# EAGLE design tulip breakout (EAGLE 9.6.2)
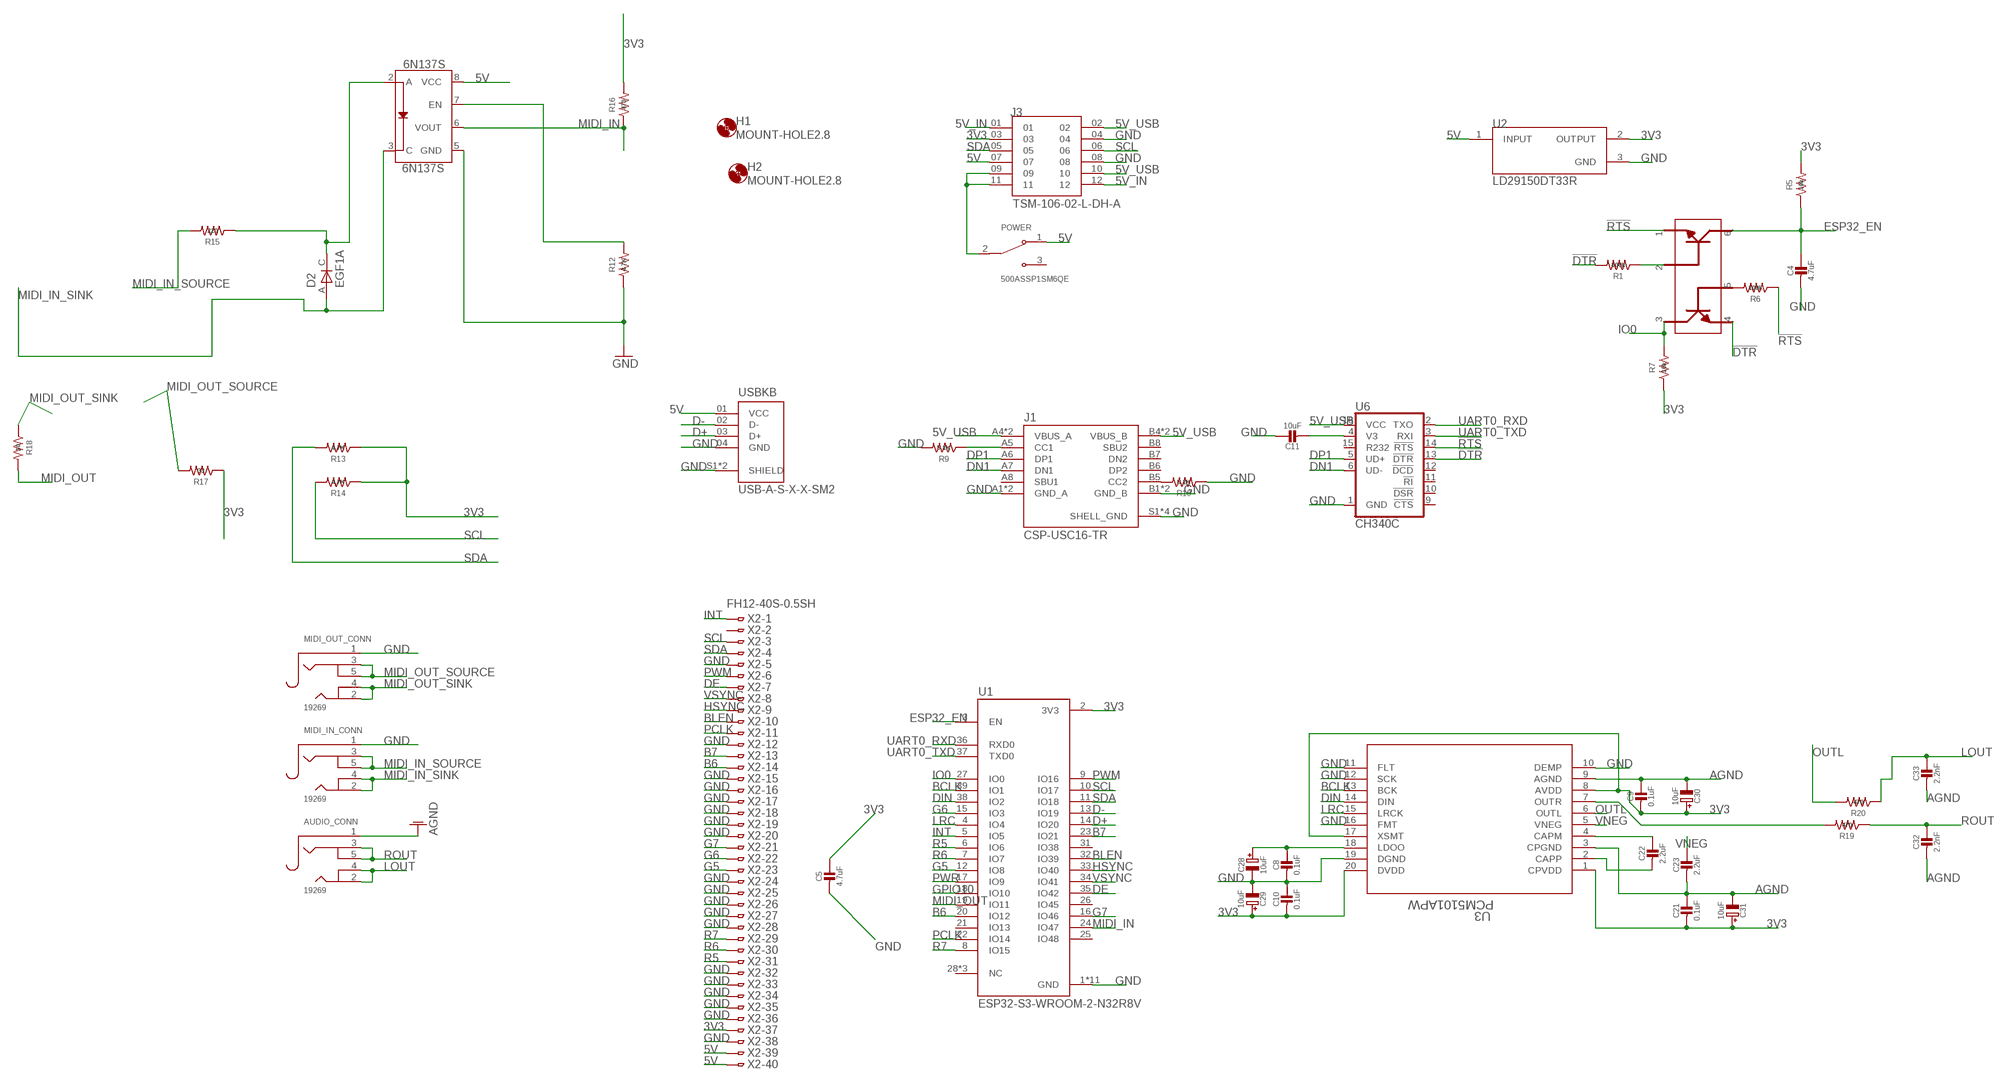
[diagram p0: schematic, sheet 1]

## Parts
6N137S  6N137S  [8-SMD]
AUDIO_CONN  19269  AUDIO_3.5MMJACK  [4UCONN_19269]
C4  4.7uF  CAP_CERAMIC0805-NOOUTLINE  [0805-NO]
C5  4.7uF  CAP_CERAMIC0805-NOOUTLINE  [0805-NO]
C8  0.1uF  CAP_CERAMIC0805-NOOUTLINE  [0805-NO]
C9  0.1uF  CAP_CERAMIC0805-NOOUTLINE  [0805-NO]
C10  0.1uF  CAP_CERAMIC0805-NOOUTLINE  [0805-NO]
C11  10uF  CAP_CERAMIC0805-NOOUTLINE  [0805-NO]
C21  0.1uF  CAP_CERAMIC0805-NOOUTLINE  [0805-NO]
C22  2.2uF  CAP_CERAMIC0805-NOOUTLINE  [0805-NO]
C23  2.2uF  CAP_CERAMIC0805-NOOUTLINE  [0805-NO]
C28  10uF  CAP_ELECTROLYTICPANASONIC_C  [PANASONIC_C]
C29  10uF  CAP_ELECTROLYTICPANASONIC_C  [PANASONIC_C]
C30  10uF  CAP_ELECTROLYTICPANASONIC_C  [PANASONIC_C]
C31  10uF  CAP_ELECTROLYTICPANASONIC_C  [PANASONIC_C]
C32  2.2nF  CAP_CERAMIC0805-NOOUTLINE  [0805-NO]
C33  2.2nF  CAP_CERAMIC0805-NOOUTLINE  [0805-NO]
D2  EGF1A  [DIOM449X264X300L114X135N]
H1  MOUNT-HOLE2.8  [2,8]
H2  MOUNT-HOLE2.8  [2,8]
J1  CSP-USC16-TR  [VALCON_CSP-USC16-TR]
J3  TSM-106-02-L-DH-A  [SAMTEC_TSM-106-02-L-DH-A]
MIDI_IN_CONN  19269  AUDIO_3.5MMJACK  [4UCONN_19269]
MIDI_OUT_CONN  19269  AUDIO_3.5MMJACK  [4UCONN_19269]
POWER  500ASSP1SM6QE  [SW_500ASSP1SM6QE]
R1  100k  R-US_R0805  [R0805]
R5  10k  R-US_R0805  [R0805]
R6  100k  R-US_R0805  [R0805]
R7  10k  R-US_R0805  [R0805]
R9  5.1K  R-US_R0805  [R0805]
R10  5.1K  R-US_R0805  [R0805]
R12  4.7K  R-US_R0805  [R0805]
R13  4.7K  R-US_R0805  [R0805]
R14  4.7K  R-US_R0805  [R0805]
R15  220  R-US_R0805  [R0805]
R16  470  R-US_R0805  [R0805]
R17  33  R-US_R0805  [R0805]
R18  10  R-US_R0805  [R0805]
R19  470  R-US_R0805  [R0805]
R20  470  R-US_R0805  [R0805]
RESET  MBT3904DW1T1G  [SOT236]
U1  ESP32-S3-WROOM-2-N32R8V  [XCVR_ESP32-S3-WROOM-2-N32R8V]
U2  LD29150DT33R  [DPAK456P972X240-3N]
U3  PCM5101APW  [PW20_TEX]
U6  CH340C  [SO016]
USBKB  USB-A-S-X-X-SM2  [SAMTEC_USB-A-S-X-X-SM2]
X2  FH12-40S-0.5SH  [FH12-40S-0.5SH]

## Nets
3V3: C5.1 C9.2 C10.2 C21.2 C29.+ C30.+ C31.+ J3.03 R5.2 R7.1 R13.1 R14.1 R16.2 R17.1 U1.2(3V3) U2.2(OUTPUT) U3.1(CPVDD) U3.8(AVDD) U3.17(XSMT) U3.20(DVDD) X2.37
5V: 6N137S.8(VCC) J3.07 POWER.1(NC) U2.1(INPUT) USBKB.01(VCC) X2.39 X2.40
5V_IN: J3.01 J3.12
5V_USB: J1.A4(VBUS_A) J1.A9(VBUS_A) J1.B4(VBUS_B) J1.B9(VBUS_B) J3.02 J3.10 U6.16(VCC)
!DTR: R1.2 RESET.4 U6.13(!DTR)
!RTS: R6.1 RESET.1 U6.14(!RTS)
AGND: AUDIO_CONN.1 C9.1 C21.1 C23.2 C30.- C31.- C32.2 C33.2 U3.3(CPGND) U3.9(AGND)
B6: U1.20(IO12) X2.14
B7: U1.23(IO21) X2.13
BCLK: U1.39(IO1) U3.13(BCK)
BLEN: U1.32(IO39) X2.10
D+: U1.14(IO20) USBKB.03(D+)
D-: U1.13(IO19) USBKB.02(D-)
DE: U1.35(IO42) X2.7
DIN: U1.38(IO2) U3.14(DIN)
DN1: J1.A7(DN1) U6.6(UD-)
DP1: J1.A6(DP1) U6.5(UD+)
ESP32_EN: C4.1 R5.1 RESET.6 U1.3(EN)
G5: U1.12(IO8) X2.23
G6: U1.15(IO3) X2.22
G7: U1.16(IO46) X2.21
GND: 6N137S.5(GND) C4.2 C5.2 C8.2 C10.1 C11.1 C28.- C29.- J1.A1(GND_A) J1.A12(GND_A) J1.B1(GND_B) J1.B12(GND_B) J1.S1(SHELL_GND) J1.S2(SHELL_GND) J1.S3(SHELL_GND) J1.S4(SHELL_GND) J3.04 J3.08 MIDI_IN_CONN.1 MIDI_OUT_CONN.1 R9.2 R10.1 R12.1 U1.1(GND) U1.40(GND) U1.41_1(GND) U1.41_2(GND) U1.41_3(GND) U1.41_4(GND) U1.41_5(GND) U1.41_6(GND) U1.41_7(GND) U1.41_8(GND) U1.41_9(GND) U2.3(GND) U3.10(DEMP) U3.11(FLT) U3.12(SCK) U3.16(FMT) U3.19(DGND) U6.1(GND) USBKB.04(GND) USBKB.S1(SHIELD) USBKB.S2(SHIELD) X2.5 X2.12 X2.15 X2.16 X2.17 X2.18 X2.19 X2.20 X2.24 X2.25 X2.26 X2.27 X2.28 X2.32 X2.33 X2.34 X2.35 X2.36 X2.38
GPIO10: U1.18(IO10)
HSYNC: U1.33(IO40) X2.9
INT: U1.5(IO5) X2.1
IO0: R7.2 RESET.3 U1.27(IO0)
LOUT: AUDIO_CONN.2 AUDIO_CONN.4 C33.1 R20.1
LRC: U1.4(IO4) U3.15(LRCK)
MIDI_IN: 6N137S.6(VOUT) R16.1 U1.24(IO47)
MIDI_IN_SINK: 6N137S.3(C) D2.A MIDI_IN_CONN.2 MIDI_IN_CONN.4
MIDI_IN_SOURCE: MIDI_IN_CONN.3 MIDI_IN_CONN.5 R15.2
MIDI_OUT: R18.2 U1.19(IO11)
MIDI_OUT_SINK: MIDI_OUT_CONN.2 MIDI_OUT_CONN.4 R18.1
MIDI_OUT_SOURCE: MIDI_OUT_CONN.3 MIDI_OUT_CONN.5 R17.2
N$1: R1.1 RESET.2
N$2: R6.2 RESET.5
N$3: J1.B5(CC2) R10.2
N$7: C8.1 C28.+ U3.18(LDOO)
N$8: R19.2 U3.7(OUTR)
N$10: J3.09 J3.11 POWER.2(COM)
N$16: C22.1 U3.4(CAPM)
N$18: C22.2 U3.2(CAPP)
N$30: 6N137S.2(A) D2.C R15.1
N$32: 6N137S.7(EN) R12.2
N$38: C11.2 U6.4(V3)
N$42: J1.A5(CC1) R9.1
OUTL: R20.2 U3.6(OUTL)
PCLK: U1.22(IO14) X2.11
PWM: U1.9(IO16) X2.6
PWR: U1.17(IO9)
R5: U1.6(IO6) X2.31
R6: U1.7(IO7) X2.30
R7: U1.8(IO15) X2.29
ROUT: AUDIO_CONN.3 AUDIO_CONN.5 C32.1 R19.1
SCL: J3.06 R14.2 U1.10(IO17) X2.3
SDA: J3.05 R13.2 U1.11(IO18) X2.4
UART0_RXD: U1.36(RXD0) U6.2(TXO)
UART0_TXD: U1.37(TXD0) U6.3(RXI)
VNEG: C23.1 U3.5(VNEG)
VSYNC: U1.34(IO41) X2.8
Unconnected: J1.A8(SBU1) J1.B6(DP2) J1.B7(DN2) J1.B8(SBU2) POWER.3(NO) U1.21(IO13) U1.25(IO48) U1.26(IO45) U1.28(NC) U1.29(NC) U1.30(NC) U1.31(IO38) U6.9(!CTS) U6.10(!DSR) U6.11(!RI) U6.12(!DCD) U6.15(R232) X2.2

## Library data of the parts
6N137S = 6N137S:6N137S: Lite-On 6N137 - High Speed Opto Isolator Opto isolator capable of data rates up to 10MBd Check availability; AVAILABILITY: In Stock; DESCRIPTION: Logic Output Optoisolator 15MBd Open Collector 5000Vrms 1 Channel 10kV/µs CMTI 8-SMD; MF: Lite-On Inc.; MP: 6N137S; PACKAGE: SMD-8 Lite-On Inc.; PRICE: None; PURCHASE-URL: https://pricing.snapeda.com/search/part/6N137S/?ref=eda
AUDIO_CONN MIDI_IN_CONN MIDI_OUT_CONN = microbuilder:AUDIO_3.5MMJACK: 3.5MM Audio Jack These are normally connected as follows, from left-to right on the schematic symbol above: Tip: Left Audio Inner Ring: Right Audio Shell: Common/GND
C4 C5 C8-C11 C21-C23 C32 C33 = microbuilder:CAP_CERAMIC: Ceramic Capacitors
C28-C31 = microbuilder:CAP_ELECTROLYTIC: Electrolytic Capacitors
D2 = EGF1A:EGF1A: EGF1A Series 1 A 100 V 50 ns Surface Mount Fast Recovery Rectifier - DO-214AC Check availability; AVAILABILITY: In Stock; DESCRIPTION: Diode Standard 50 V 1A Surface Mount DO-214AC (SMA); MF: ON Semiconductor; MP: EGF1A; PACKAGE: SMA-2 ON Semiconductor; PRICE: None; PURCHASE-URL: https://pricing.snapeda.com/search/part/EGF1A/?ref=eda
H1 H2 = holes:MOUNT-HOLE: MOUNTING HOLE with drill center marker
J1 = CSP-USC16-TR:CSP-USC16-TR: CSP-USC16-TR Valcon USB Type C Surface Mount PCB Socket Check availability; AVAILABILITY: In Stock; DESCRIPTION: CSP-USC16-TR Valcon USB Type C Surface Mount PCB Socket; MF: Valcon; MP: CSP-USC16-TR; PACKAGE: None; PRICE: None; PURCHASE-URL: https://pricing.snapeda.com/search/part/CSP-USC16-TR/?ref=eda
J3 = TSM-106-02-L-DH-A:TSM-106-02-L-DH-A; DESCRIPTION: Connector Header Surface Mount, Right Angle 12 position 0.100 (2.54mm); DIGI-KEY_PART_NUMBER: 612-TSM-106-02-L-DH-A-ND; MF: Samtec; MP: TSM-106-02-L-DH-A; PACKAGE: None; PURCHASE-URL: https://pricing.snapeda.com/search/part/TSM-106-02-L-DH-A/?ref=eda
POWER = 500ASSP1SM6QE:500ASSP1SM6QE; DESCRIPTION: Slide Switch SPDT Surface Mount, Right Angle; DIGI-KEY_PART_NUMBER: EG5810TR-ND; MF: E-Switch; MP: 500ASSP1SM6QE; PACKAGE: None; PURCHASE-URL: https://pricing.snapeda.com/search/part/500ASSP1SM6QE/?ref=eda
R1 R5-R7 R9 R10 R12-R20 = adafruit:R-US_: RESISTOR, American symbol
RESET = MBT3904DW1T1G:MBT3904DW1T1G: Check availability; AVAILABILITY: In Stock; DESCRIPTION: Bipolar (BJT) Transistor Array 2 NPN (Dual) 40V 200mA 300MHz 150mW Surface Mount SC-88/SC70-6/SOT-363; MF: ON Semiconductor; MP: MBT3904DW1T1G; PACKAGE: SC-88-6 ON Semiconductor; PRICE: None; PURCHASE-URL: https://pricing.snapeda.com/search/part/MBT3904DW1T1G/?ref=eda
U1 = ESP32-S3-WROOM-2-N32R8V:ESP32-S3-WROOM-2-N32R8V: Check availability; AVAILABILITY: In Stock; DESCRIPTION: Bluetooth, WiFi 802.11b/g/n, Bluetooth v5.0 Transceiver Module 2.4GHz PCB Trace Surface Mount; MF: Espressif Systems; MP: ESP32-S3-WROOM-2-N32R8V; PACKAGE: Package; PRICE: None; PURCHASE-URL: https://pricing.snapeda.com/search/part/ESP32-S3-WROOM-2-N32R8V/?ref=eda
U2 = LD29150DT33R:LD29150DT33R: LD29150 Series 1.5 A 3.3 V Fixed Output SMT LDO Voltage Regulator - TO-252; DESCRIPTION: Linear Voltage Regulator IC Positive Fixed 1 Output 1.5A DPAK; DIGI-KEY_PART_NUMBER: 497-1496-2-ND; MF: STMicroelectronics; MP: LD29150DT33R; PACKAGE: TO-252 STMicroelectronics; PURCHASE-URL: https://pricing.snapeda.com/search/part/LD29150DT33R/?ref=eda
U3 = pcm5101apw:PCM5101APW; COPYRIGHT: Copyright (C) 2022 Ultra Librarian. All rights reserved.; DIGI-KEY_PART_NUMBER_1: PCM5101APW-ND; MANUFACTURER_PART_NUMBER: PCM5101APW; MFR_NAME: Texas Instruments
U6 = SparkFun-IC-Comms:CH340C; PROD_ID: IC-14038
USBKB = USB-A-S-X-X-SM2:USB-A-S-X-X-SM2: USB-A (USB TYPE-A) USB 2.0 Receptacle Connector 4 Position Surface Mount, Right Angle; Through Hole Check availability; AVAILABILITY: In Stock; DESCRIPTION: USB-A (USB TYPE-A) USB 2.0 Receptacle Connector 4 Position Surface Mount, Right Angle; MF: Samtec; MP: USB-A-S-F-W-SM2-TR; PACKAGE: None; PRICE: None; PURCHASE-URL: https://pricing.snapeda.com/search/part/USB-A-S-F-W-SM2-TR/?ref=eda
X2 = con-hirose:FH12-40S-0.5S: 0.5mm Pitch Connectors For FPC/FFC Source: Data sheet; MPN: FH12-40S-0.5SH(55); OC_FARNELL: 1324556; OC_NEWARK: 34M6178

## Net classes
1 power: width 0.178 mm

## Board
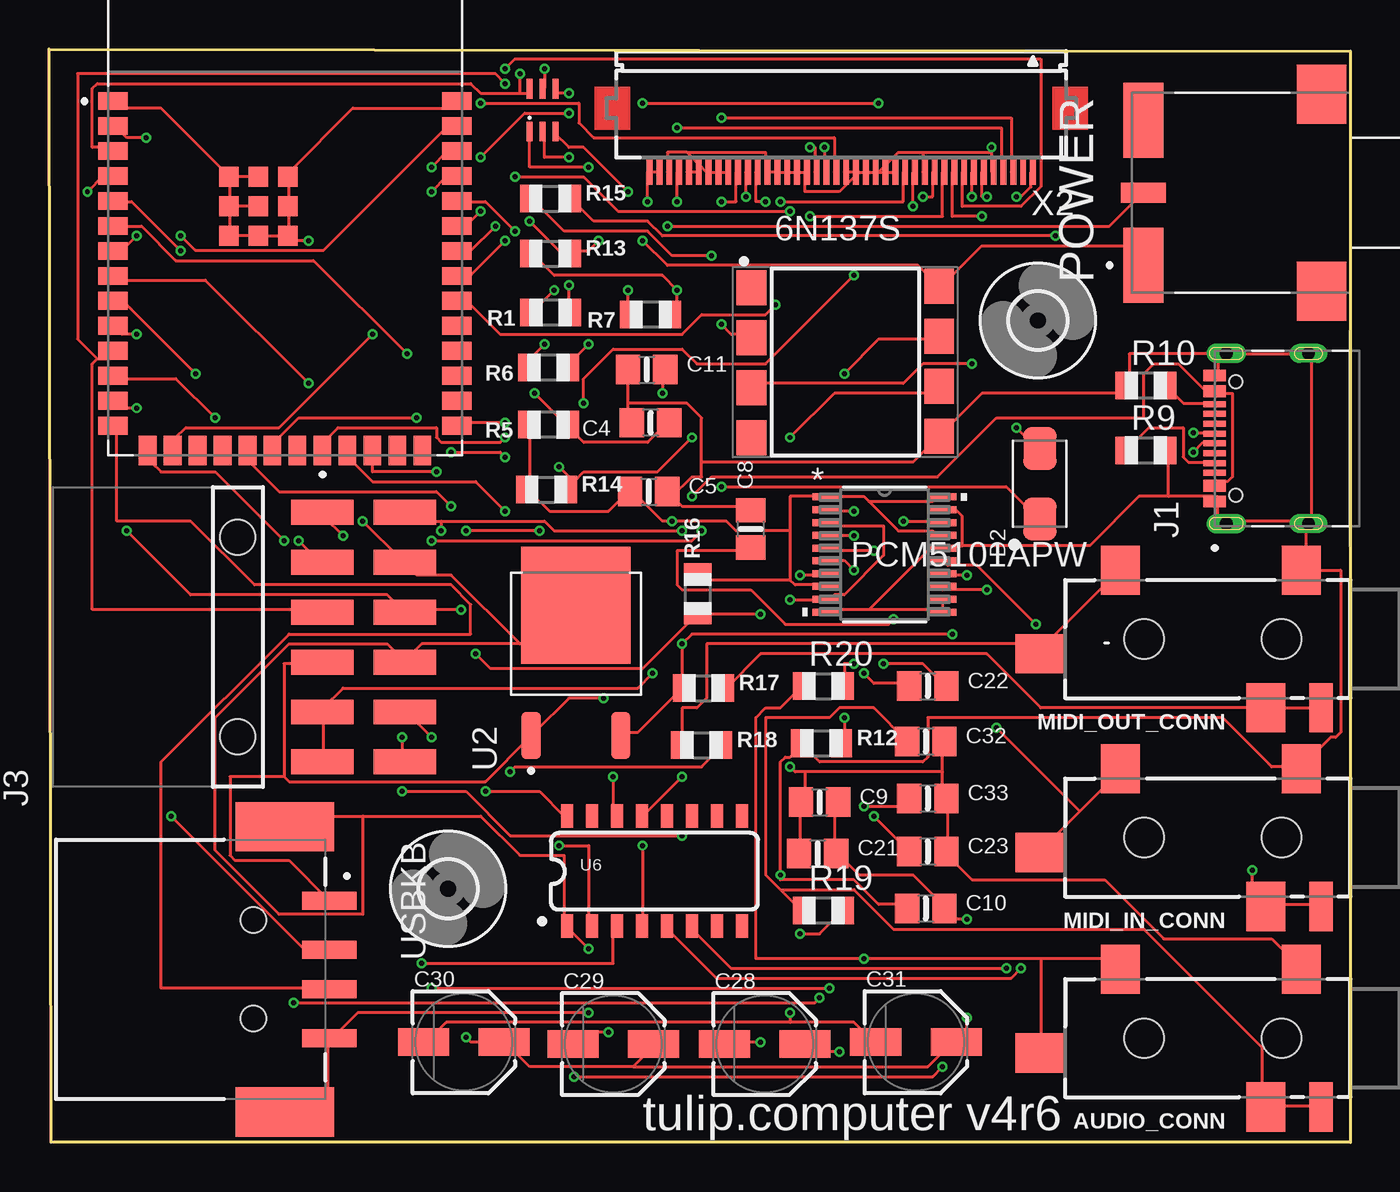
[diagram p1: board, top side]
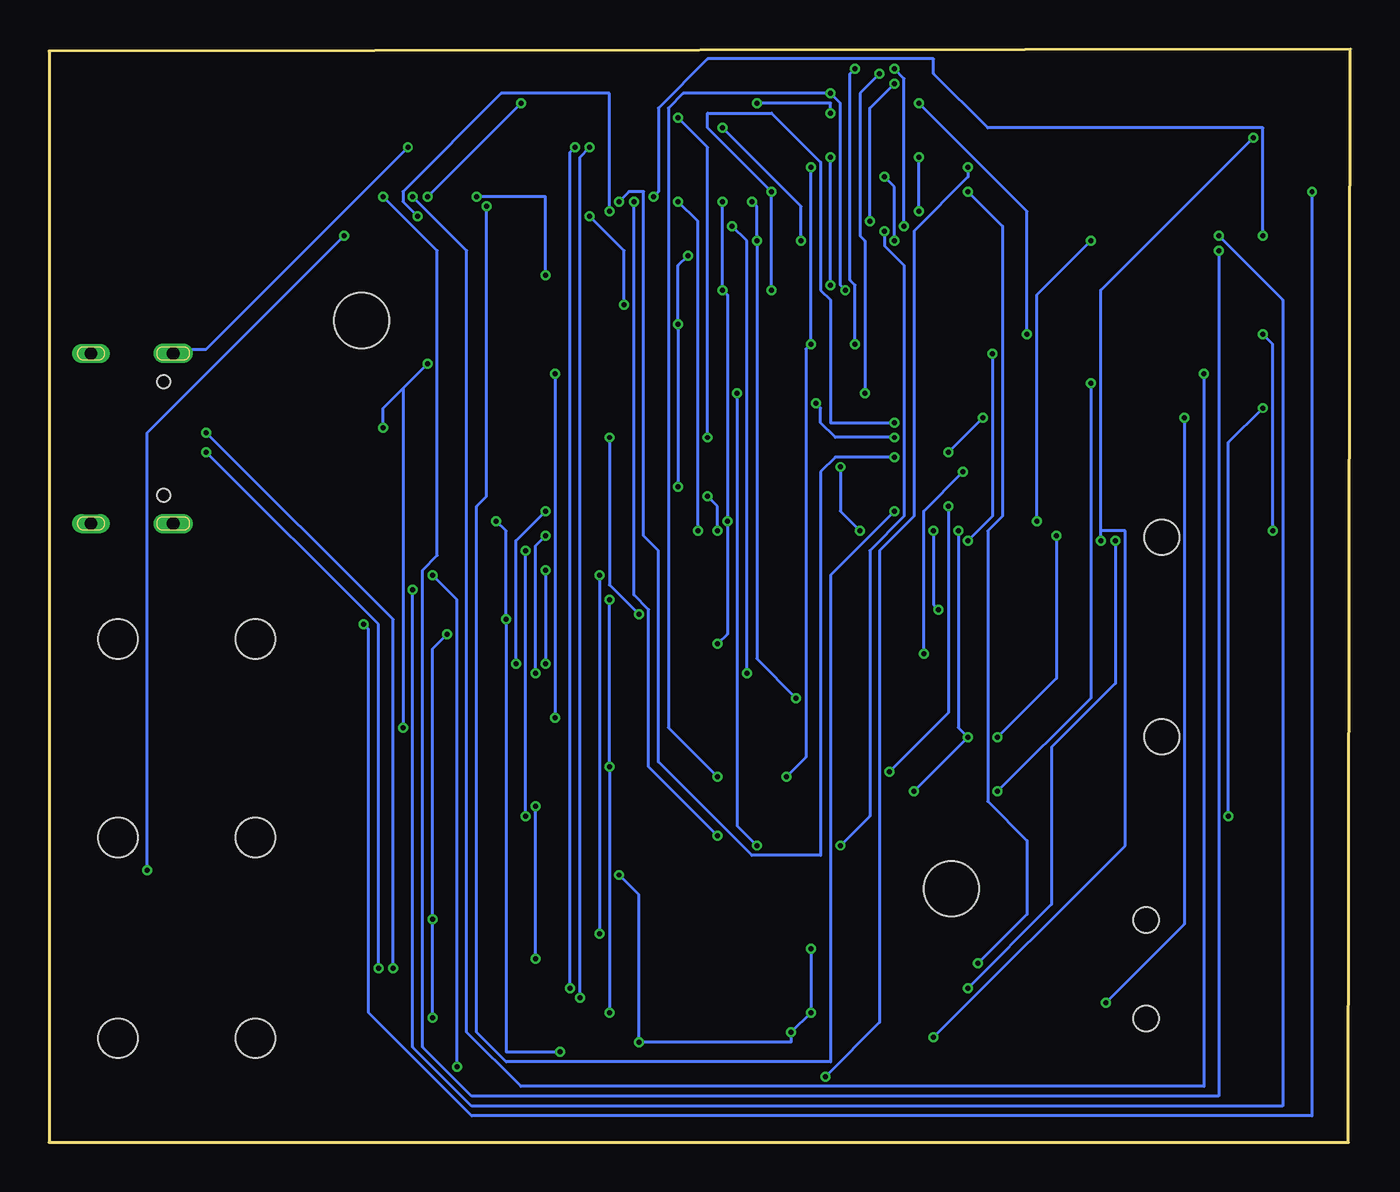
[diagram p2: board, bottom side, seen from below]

Size 66.2 x 55.6 mm. Coordinates in mm from the lower left corner, seen from the top.
Outline: 0.1,0 0,55.6 66.2,55.5 66.2,0 0.1,0
Copper layers (1*16): Top 0.035559375mm / dielectric 1.6mm / Bottom 0.035559375mm
Design rules "oshpark-2layer *": minimum track width 6mil, minimum drill 10mil, track to track 6mil, track to pad 6mil, pad to pad 6mil, via to via 6mil, smd to smd 6mil, copper to edge 0mil, drill to drill 6mil, minimum pad ring 5mil, minimum via ring 5mil, stop-mask expansion 2.5mil, vias tented up to drill 0mil, thermal gap 10mil

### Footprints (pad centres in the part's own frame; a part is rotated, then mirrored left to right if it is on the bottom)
8-SMD = smd 1.52 x 1.78: 1 -4.96,3.96; 2 -4.96,1.42; 3 -4.96,-1.12; 4 -4.96,-3.66; 5 4.58,-3.59; 6 4.58,-1.05; 7 4.58,1.49; 8 4.58,4.03
4UCONN_19269 = smd 2 x 2.5: 1 2.5,-3.5; 2 11.7,-3.5; 3 4.3,3.5 | smd 2.5 x 2: 4 15.8,0.75 | smd 1.2 x 2.5: 5 1.5,3.5 | hole 2: 3.5,0; 10.5,0
0805-NO = smd 1.24 x 1.5: 1 -0.95,0; 2 0.95,0
PANASONIC_C = smd 2.6 x 1.4: + 2.05,0; - -2.05,0
DIOM449X264X300L114X135N = smd 2.17 x 1.69: A 1.795,0; C -1.795,0
2,8 = hole 2.8: 0,0
VALCON_CSP-USC16-TR = smd 0.3 x 1.14: A1 -3.35,0; A4 -2.55,0; A5 -1.25,0; A6 -0.25,0; A7 0.25,0; A8 1.25,0; A9 2.55,0; A12 3.35,0; B1 3.05,0; B4 2.25,0; B5 1.75,0; B6 0.75,0; B7 -0.75,0; B8 -1.75,0; B9 -2.25,0; B12 -3.05,0 | drill 0.65 pad 1 long: S1 -4.325,-0.59; S2 4.325,-0.59 | drill 0.65 pad 0.9 long: S3 -4.325,-4.77; S4 4.325,-4.77 | hole 0.65: -2.89,-1.07; 2.89,-1.07
SAMTEC_TSM-106-02-L-DH-A = smd 1.27 x 3.18: 01 6.35,-4.305; 02 6.35,-8.495; 03 3.81,-4.305; 04 3.81,-8.495; 05 1.27,-4.305; 06 1.27,-8.495; 07 -1.27,-4.305; 08 -1.27,-8.495; 09 -3.81,-4.305; 10 -3.81,-8.495; 11 -6.35,-4.305; 12 -6.35,-8.495 | hole 1.78: -5.08,0; 5.08,0
SW_500ASSP1SM6QE = smd 3.81 x 2.03: 1 -3.685,4.535; 3 3.685,4.535 | smd 1.02 x 2.29: 2 0,4.535 | smd 3 x 2.5: S1 -5,-4.535; S2 5,-4.535
R0805 = smd 1.1 x 1.4: 1 -1,0; 2 1,0
SOT236 = smd 0.3 x 1: 1 -0.66,-1.09; 2 0,-1.09; 3 0.66,-1.09; 4 0.66,1.09; 5 0,1.09; 6 -0.66,1.09
XCVR_ESP32-S3-WROOM-2-N32R8V = smd 1.5 x 0.9: 1 -8.75,5.26; 2 -8.75,3.99; 3 -8.75,2.72; 4 -8.75,1.45; 5 -8.75,0.18; 6 -8.75,-1.09; 7 -8.75,-2.36; 8 -8.75,-3.63; 9 -8.75,-4.9; 10 -8.75,-6.17; 11 -8.75,-7.44; 12 -8.75,-8.71; 13 -8.75,-9.98; 14 -8.75,-11.25; 27 8.75,-11.25; 28 8.75,-9.98; 29 8.75,-8.71; 30 8.75,-7.44; 31 8.75,-6.17; 32 8.75,-4.9; 33 8.75,-3.63; 34 8.75,-2.36; 35 8.75,-1.09; 36 8.75,0.18; 37 8.75,1.45; 38 8.75,2.72; 39 8.75,3.99; 40 8.75,5.26 | smd 0.9 x 1.5: 15 -6.985,-12.5; 16 -5.715,-12.5; 17 -4.445,-12.5; 18 -3.175,-12.5; 19 -1.905,-12.5; 20 -0.635,-12.5; 21 0.635,-12.5; 22 1.905,-12.5; 23 3.175,-12.5; 24 4.445,-12.5; 25 5.715,-12.5; 26 6.985,-12.5 | smd 1 x 1: 41_1 -1.36,-0.09; 41_2 -2.86,-0.09; 41_3 0.14,-0.09; 41_4 -2.86,-1.59; 41_5 -1.36,-1.59; 41_6 0.14,-1.59; 41_7 -2.86,1.41; 41_8 -1.36,1.41; 41_9 0.14,1.41
DPAK456P972X240-3N = smd 2.4 x 0.98: 1 -4.2,2.28; 2 -4.2,-2.28 | smd 5.96 x 5.57: 3 2.42,0
PW20_TEX = smd 1.473 x 0.356: 1 -2.921,2.925; 2 -2.921,2.275; 3 -2.921,1.625; 4 -2.921,0.975; 5 -2.921,0.325; 6 -2.921,-0.325; 7 -2.921,-0.975; 8 -2.921,-1.625; 9 -2.921,-2.275; 10 -2.921,-2.925; 11 2.921,-2.925; 12 2.921,-2.275; 13 2.921,-1.625; 14 2.921,-0.975; 15 2.921,-0.325; 16 2.921,0.325; 17 2.921,0.975; 18 2.921,1.625; 19 2.921,2.275; 20 2.921,2.925
SO016 = smd 0.6 x 1.2: 1 -4.445,-2.8; 2 -3.175,-2.8; 3 -1.905,-2.8; 4 -0.635,-2.8; 5 0.635,-2.8; 6 1.905,-2.8; 7 3.175,-2.8; 8 4.445,-2.8; 9 4.445,2.8; 10 3.175,2.8; 11 1.905,2.8; 12 0.635,2.8; 13 -0.635,2.8; 14 -1.905,2.8; 15 -3.175,2.8; 16 -4.445,2.8
SAMTEC_USB-A-S-X-X-SM2 = smd 0.9 x 2.8: 01 -3.5,3.85; 02 -1,3.85; 03 1,3.85; 04 3.5,3.85 | smd 2.5 x 5: S1 -7.25,1.6; S2 7.25,1.6 | hole 1.3: -2.5,0; 2.5,0
FH12-40S-0.5SH = smd 0.3 x 1.3: 1 -9.75,3.25; 2 -9.25,3.25; 3 -8.75,3.25; 4 -8.25,3.25; 5 -7.75,3.25; 6 -7.25,3.25; 7 -6.75,3.25; 8 -6.25,3.25; 9 -5.75,3.25; 10 -5.25,3.25; 11 -4.75,3.25; 12 -4.25,3.25; 13 -3.75,3.25; 14 -3.25,3.25; 15 -2.75,3.25; 16 -2.25,3.25; 17 -1.75,3.25; 18 -1.25,3.25; 19 -0.75,3.25; 20 -0.25,3.25; 21 0.25,3.25; 22 0.75,3.25; 23 1.25,3.25; 24 1.75,3.25; 25 2.25,3.25; 26 2.75,3.25; 27 3.25,3.25; 28 3.75,3.25; 29 4.25,3.25; 30 4.75,3.25; 31 5.25,3.25; 32 5.75,3.25; 33 6.25,3.25; 34 6.75,3.25; 35 7.25,3.25; 36 7.75,3.25; 37 8.25,3.25; 38 8.75,3.25; 39 9.25,3.25; 40 9.75,3.25

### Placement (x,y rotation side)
6N137S  40.7,39.5 0 top
AUDIO_CONN  66.2,5.3 180 top
C4  30.6,36.6 180 top
C5  30.5,33.1 0 top
C8  35.7,31.2 90 top
C9  39.2,17.3 0 top
C10  44.6,11.9 0 top
C11  30.4,39.3 0 top
C21  39.1,14.7 0 top
C22  44.7,23.2 0 top
C23  44.7,14.8 0 top
C28  36.4,5 0 top
C29  28.7,5 0 top
C30  21.1,5.1 0 top
C31  44.1,5.1 0 top
C32  44.6,20.4 0 top
C33  44.7,17.5 0 top
D2  50.4,33.5 90 top
H1  20.3,12.9 0 top
H2  50.3,41.8 0 top
J1  59.3,35.8 90 top
J3  9.6,25.7 90 top
MIDI_IN_CONN  66.2,15.5 180 top
MIDI_OUT_CONN  66.2,25.6 180 top
POWER  60.2,48.3 90 top
R1  25.5,42.2 180 top
R5  25.4,36.5 180 top
R6  25.4,39.4 180 top
R7  30.6,42.1 180 top
R9  55.8,35.2 0 top
R10  55.8,38.5 0 top
R12  39.3,20.3 0 top
R13  25.5,45.2 0 top
R14  25.3,33.2 0 top
R15  25.5,48 0 top
R16  33,27.9 90 top
R17  33.3,23.1 0 top
R18  33.2,20.2 0 top
R19  39.4,11.8 0 top
R20  39.4,23.2 0 top
RESET  25.1,52.5 0 top
U1  12,47.7 0 top
U2  26.8,24.9 90 top
U3  42.5,29.9 0 top
U6  30.8,13.8 0 top
USBKB  10.4,8.8 270 top
X2  40.3,52.6 180 top

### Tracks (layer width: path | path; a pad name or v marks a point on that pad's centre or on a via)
3V3  (via drill 0.25)
  Top 0.152: R5.2 24.45,36.35 24.45,33.35 R14.1 24.45,33.1 25.45,32.1 28.45,32.1 29.45,33.1 C5.1 29.7,33.1 31.2,31.6 v31.7,31.6 34.45,31.6 34.95,31.1 37.7,31.1 | 37.7,28.6 33.45,28.6 33.2,28.85 R16.2 | 37.7,28.6 37.95,28.35 39.45,28.35 U3.8 | 41.7,32.6 41.45,32.85 39.7,32.85 U3.1 39.45,32.85 37.7,32.85 37.7,31.1 | 41.7,32.6 43.2,31.1 44.95,31.1 45.2,30.85 U3.17 | 41.7,32.6 44.95,32.6 45.2,32.85 U3.20 | 37.7,31.1 37.7,28.6 | 32.2,23.1 29.95,20.85 29.2,20.85 U2.2 | v31.95,47.85 31.95,49.35 X2.37 | R7.1 31.95,42.1 v31.95,43.35 31.2,44.1 25.7,44.1 24.7,45.1 R13.1 | 32.2,23.1 v32.2,25.35 32.7,25.85 v45.95,25.85 | 32.2,23.1 R17.1 | v4.95,51.1 3.95,51.1 3.45,51.6 U1.2 | v12.7,30.6 13.7,29.6 J3.03 | C9.2 39.95,17.1 39.95,14.85 C21.2 40.2,14.6 41.2,13.6 43.95,13.6 45.45,12.1 C10.2 45.7,11.85 46.2,11.35 v46.7,11.35 | 29.7,3.85 24.45,3.85 23.2,5.1 C30.+ 21.45,5.1 v21.2,5.35 | 29.7,3.85 30.7,4.85 C29.+ | 29.7,3.85 44.7,3.85 45.95,5.1 C31.+ 46.7,5.1 v46.7,6.35
  Bottom 0.152: v31.95,47.85 v31.95,43.35 31.7,43.1 v31.7,31.6 31.7,25.85 v32.2,25.35 | v4.95,51.1 12.7,43.35 12.7,31.1 | v12.7,30.6 12.7,31.1 | v46.7,6.35 v46.7,11.35 46.7,25.1 v45.95,25.85 | 12.7,31.1 11.45,31.1 11.45,15.1 v21.2,5.35
5V  (via drill 0.25)
  Top 0.152: 11.95,18.6 12.2,18.35 22.2,18.35 24.45,20.6 U2.1 24.7,20.85 26.45,22.6 v28.2,22.6 | 11.95,18.6 11.95,24.35 13.7,24.35 J3.07 | USBKB.01 12.2,14.35 9.45,14.35 9.2,14.6 9.2,18.6 11.95,18.6 | X2.39 X2.40 30.45,49.35 v30.45,47.85 | v30.2,45.85 31.45,44.6 44.2,44.6 45.2,43.6 6N137S.8 45.45,43.6 47.45,45.6 54.7,45.6 55.45,44.85 POWER.1
  Bottom 0.152: v30.45,47.85 30.2,47.6 v30.2,45.85 30.2,24.6 v28.2,22.6
5V_IN  (via drill 0.25)
  Top 0.152: v17.95,20.6 17.95,19.35 J3.12 | v14.95,30.85 13.95,31.85 J3.01
  Bottom 0.152: v17.95,20.6 14.95,23.6 v14.95,30.85
5V_USB  (via drill 0.25)
  Top 0.152: v22.2,17.85 24.95,17.85 26.2,16.6 U6.16 | v19.45,20.6 18.2,21.85 J3.10 | 59.45,33.6 59.45,33.35 J1.A4 | 59.45,38.1 59.45,38.35 J1.A9 58.7,38.35 57.45,39.6 56.2,39.6 55.7,39.1 55.7,36.85 48.2,36.85 45.2,33.85 33.7,33.85 v32.7,32.85 | 59.45,33.6 59.95,33.6 60.2,33.85 60.2,38.1 59.45,38.1 | 59.45,33.6 J1.B9 | 59.45,38.1 J1.B4 | v32.2,31.1 25.7,31.1 25.2,31.6 19.95,31.6 | 19.95,31.6 18.45,31.6 18.2,31.85 J3.02 | 19.95,31.6 v19.95,31.1
  Bottom 0.152: v22.2,17.85 v19.45,20.6 19.95,21.1 v19.95,31.1 | v32.7,32.85 32.2,32.35 v32.2,31.1
!DTR  (via drill 0.25)
  Top 0.152: v26.45,53.35 25.7,53.35 RESET.4 | v25.7,43.35 24.7,42.35 R1.2 | v32.2,18.6 30.2,16.6 U6.13
  Bottom 0.152: v25.7,43.35 25.95,43.6 25.95,52.85 v26.45,53.35 33.95,53.35 34.7,52.6 34.7,21.1 v32.2,18.6
!RTS  (via drill 0.25)
  Top 0.152: v27.45,49.6 24.45,49.6 24.45,51.35 RESET.1 | v27.45,40.6 26.45,39.6 R6.1 | v28.7,18.6 28.7,16.6 U6.14
  Bottom 0.152: v27.45,49.6 v27.45,40.6 27.7,40.35 27.7,19.6 v28.7,18.6
AGND  (via drill 0.25)
  Top 0.152: 37.7,6.1 40.95,6.1 41.95,5.1 C31.- | 37.7,6.1 20.2,6.1 19.2,5.1 C30.- | U3.3 39.7,31.35 42.45,31.35 42.45,29.85 40.45,27.85 39.95,27.85 39.7,27.6 U3.9 39.45,27.6 v37.7,27.6 | C21.1 38.2,14.85 38.2,17.1 C9.1 38.45,17.35 38.45,18.85 | 45.45,18.85 45.45,17.6 C33.2 45.7,17.35 45.7,14.85 C23.2 45.7,14.6 46.95,13.35 53.7,13.35 56.7,10.35 62.2,10.35 63.7,8.85 AUDIO_CONN.1 | 45.45,18.85 45.45,20.35 C32.2 | 45.45,18.85 38.45,18.85 | v37.7,19.1 37.95,18.85 38.45,18.85 | v37.7,6.6 37.7,6.1
  Bottom 0.152: v37.7,27.6 v37.7,19.1 v37.7,6.6
B6  (via drill 0.25)
  Top 0.152: v37.2,47.85 43.45,47.85 43.45,49.35 X2.14 | v23.2,34.85 22.95,35.1 v20.45,35.1 | v18.7,36.85 12.7,36.85 11.2,35.35 U1.20
  Bottom 0.152: v37.2,47.85 36.7,48.35 35.95,48.35 35.95,30.85 35.2,30.1 35.2,19.35 30.45,14.6 26.95,14.6 26.95,34.1 26.2,34.85 v23.2,34.85 | v18.7,36.85 v20.45,35.1
B7  (via drill 0.25)
  Top 0.152: v43.95,47.6 43.95,49.35 X2.13 | v23.2,32.1 21.7,33.6 16.45,33.6 14.95,35.1 U1.23
  Bottom 0.152: v43.95,47.6 43.95,32.85 44.45,32.35 44.45,5.6 42.95,4.1 26.45,4.1 26.45,28.85 v23.2,32.1
BCLK  (via drill 0.25)
  Top 0.152: v47.7,28.1 45.45,28.1 U3.13 | v6.7,46.1 7.45,45.35 13.95,45.35 20.2,51.6 20.7,51.6 U1.39
  Bottom 0.152: v47.7,28.1 47.7,4.85 44.7,1.85 3.45,1.85 3.45,42.85 v6.7,46.1
BLEN  (via drill 0.25)
  Top 0.152: v38.7,47.1 45.45,47.1 45.45,49.35 X2.10 | v36.95,42.6 36.45,42.1 33.2,42.1 32.2,41.1 22.95,41.1 21.45,42.6 20.95,42.6 U1.32
  Bottom 0.152: v38.7,47.1 36.95,45.35 v36.95,42.6
D+
  Top 0.152: U1.14 3.45,36.35 3.45,31.6 7.2,31.6 10.45,28.35 20.45,28.35 21.45,27.35 21.45,25.85 12.2,25.85 5.7,19.35 5.7,7.85 14.2,7.85 USBKB.03
D-  (via drill 0.25)
  Top 0.152: v4.45,37.35 3.7,37.35 3.45,37.6 U1.13 | v6.2,16.6 12.95,9.85 14.2,9.85 USBKB.02
  Bottom 0.152: v4.45,37.35 6.2,35.6 v6.2,16.6
DE  (via drill 0.25)
  Top 0.152: v46.95,48.1 46.95,49.35 X2.7 | v30.2,52.85 v42.2,52.85 | v26.45,52.35 24.2,52.35 v21.95,50.1 | v21.95,47.35 21.45,46.85 20.95,46.85 U1.35
  Bottom 0.152: v42.2,52.85 v46.95,48.1 | v30.2,52.85 26.45,52.85 v26.45,52.35 | v21.95,47.35 v21.95,50.1
DIN  (via drill 0.25)
  Top 0.152: v46.7,28.85 45.45,28.85 U3.14 | v45.45,3.85 44.95,3.35 v26.7,3.35 | v19.45,49.6 20.2,50.35 20.7,50.35 U1.38
  Bottom 0.152: v46.7,28.85 45.45,27.6 v45.45,3.85 | v26.7,3.35 23.95,6.1 23.95,30.1 22.2,31.85 22.2,46.35 19.45,49.1 v19.45,49.6
DN1  (via drill 0.25)
  Top 0.152: v58.2,36.1 59.2,36.1 J1.A7 | v48.7,8.85 34.7,8.85 32.7,10.85 U6.6
  Bottom 0.152: v58.2,36.1 48.7,26.6 v48.7,8.85
DP1  (via drill 0.25)
  Top 0.152: v58.2,35.1 58.7,35.6 59.2,35.6 J1.A6 | v49.45,8.85 48.95,8.35 33.95,8.35 31.45,10.85 U6.5
  Bottom 0.152: v58.2,35.1 49.45,26.35 v49.45,8.85
ESP32_EN  (via drill 0.25)
  Top 0.152: C4.1 31.45,36.6 30.45,35.6 27.2,35.6 26.45,36.35 R5.1 26.2,36.6 v24.7,38.1 | 23.95,53.35 21.95,53.35 21.45,53.85 2.45,53.85 2.2,53.6 2.2,50.6 3.2,50.6 U1.3 | 23.95,53.35 24.45,53.35 RESET.6 | 23.95,53.35 v23.95,54.35
  Bottom 0.152: v24.7,38.1 24.7,45.85 24.95,46.1 24.95,53.35 v23.95,54.35
G5  (via drill 0.25)
  Top 0.152: v38.7,50.6 38.95,50.6 38.95,49.35 X2.23 | v39.2,7.35 38.95,7.1 v12.45,7.1 | v8.45,36.85 6.45,38.85 3.45,38.85 U1.12
  Bottom 0.152: v38.7,50.6 39.2,50.1 v39.2,7.35 | v12.45,7.1 8.45,11.1 v8.45,36.85
G6  (via drill 0.25)
  Top 0.152: v39.45,50.6 39.45,49.35 X2.22 | v19.45,7.85 v39.7,7.85 | v11.95,30.6 8.45,34.1 5.7,34.1 5.2,34.6 5.2,35.1 U1.15
  Bottom 0.152: v39.45,50.6 39.7,50.35 v39.7,7.85 | v19.45,7.85 15.2,12.1 15.2,20.1 11.95,23.35 v11.95,30.6
G7  (via drill 0.25)
  Top 0.152: v21.95,52.85 26.95,52.85 26.95,51.85 27.7,51.1 39.95,51.1 39.95,49.35 X2.21 | v16.45,41.1 11.7,36.35 6.95,36.35 6.45,35.85 6.45,35.35 U1.16
  Bottom 0.152: v21.95,52.85 16.45,47.35 v16.45,41.1
GND  (via drill 0.25)
  Top 0.152: C10.1 43.45,12.1 42.2,12.1 40.95,13.35 37.2,13.35 v37.2,13.6 37.2,19.35 37.45,19.6 37.7,19.6 38.2,20.1 R12.1 38.45,20.1 39.2,19.35 44.45,19.35 44.7,19.6 44.7,21.6 59.7,21.6 62.2,19.1 63.7,19.1 | U3.12 45.45,27.6 45.45,27.1 U3.11 45.2,27.1 41.7,27.1 | 41.7,27.1 39.7,27.1 U3.10 | 41.7,27.1 44.7,30.1 45.2,30.1 U3.16 45.45,30.35 46.45,30.35 | 46.45,30.35 46.45,31.85 46.2,32.1 45.45,32.1 U3.19 | 59.45,32.35 59.45,32.85 J1.B12 59.2,32.85 56.95,32.85 | 59.45,32.35 59.45,31.6 59.7,31.6 J1.S1 59.95,31.6 63.95,31.6 J1.S3 | 59.45,32.35 J1.A1 | 56.95,32.85 56.95,35.1 R9.2 | 63.95,29.1 63.95,31.35 J1.S3 | 63.7,19.1 65.2,20.6 65.45,20.6 65.7,20.85 65.7,29.1 63.95,29.1 | 63.95,29.1 MIDI_OUT_CONN.1 | 46.45,30.35 52.95,30.35 55.45,32.85 56.95,32.85 | 63.7,19.1 MIDI_IN_CONN.1 | 38.45,49.35 X2.25 37.95,49.35 X2.26 37.45,49.35 X2.27 36.95,49.35 X2.28 36.45,49.35 36.45,50.35 32.45,50.35 | 32.95,49.35 X2.36 32.45,49.35 | 32.45,50.35 31.45,50.35 31.45,49.35 X2.38 | 33.2,49.6 33.45,49.35 X2.34 33.95,49.35 X2.33 X2.32 | 33.2,49.6 32.45,50.35 | 33.2,49.6 32.95,49.35 | 32.95,49.35 X2.35 | 40.45,49.35 X2.20 40.95,49.35 X2.19 41.2,49.35 | 41.2,49.35 41.45,49.35 X2.18 41.95,49.35 X2.17 42.2,49.35 | 42.2,49.35 42.45,49.35 X2.16 X2.15 | 44.45,50.35 44.45,49.35 X2.12 | 44.45,50.35 43.2,50.35 42.2,49.35 | 47.95,50.35 47.95,49.35 X2.5 | 44.45,50.35 47.95,50.35 | 38.45,49.35 38.45,48.35 40.2,48.35 41.2,49.35 | 38.45,49.35 X2.24 | 29.45,37.6 29.45,36.6 C4.2 | 29.45,37.6 C11.1 | 31.7,32.85 32.2,32.35 35.7,32.35 C8.2 | 29.45,37.6 32.45,37.6 33.2,36.85 33.2,34.6 | 33.2,34.6 33.2,33.85 32.7,33.85 31.7,32.85 | 31.7,32.85 C5.2
  Top 0.152: 59.45,39.1 59.45,38.85 J1.B1 | 59.45,40.1 59.45,39.1 | 59.45,40.1 59.7,40.1 J1.S2 | 59.45,39.1 J1.A12 | 59.45,40.1 54.95,40.1 54.95,38.6 R10.1 54.7,38.35 54.45,38.1 47.45,38.1 45.45,36.1 6N137S.5 45.2,35.85 43.95,34.6 33.2,34.6 | 59.45,40.1 J1.S2 | J1.S2 59.95,40.1 63.95,40.1 J1.S4 64.2,40.1 64.2,31.6 J1.S3 | v47.95,50.6 47.95,50.35 | 9.2,49.1 10.45,49.1 U1.41_8 | 9.2,47.6 10.45,47.6 U1.41_1 | U1.41_6 11.95,46.1 10.7,46.1 U1.41_5 10.45,46.1 9.2,46.1 U1.41_4 9.2,46.35 9.2,47.6 | U1.41_6 12.2,46.35 12.2,47.6 U1.41_3 12.2,47.85 12.2,49.1 U1.41_9 12.2,49.35 15.45,52.6 20.45,52.6 20.7,52.85 U1.40 | 9.2,47.6 U1.41_2 9.2,47.85 9.2,49.1 | 9.2,49.1 U1.41_7 8.95,49.35 5.7,52.6 3.7,52.6 3.45,52.85 U1.1 | 23.95,25.35 24.95,25.35 26.7,27.1 U2.3 | 23.95,25.35 18.95,25.35 18.2,24.6 J3.08 17.95,24.6 17.2,25.35 12.2,25.35 8.45,21.6 8.45,14.85 11.7,11.6 15.95,11.6 15.95,16.6 | 23.95,25.35 20.45,28.85 18.7,28.85 18.2,29.35 J3.04 17.95,29.6 v15.95,31.6 | USBKB.S2 12.2,1.6 14.2,1.6 14.2,5.1 USBKB.04 14.45,5.35 15.7,6.6 v27.45,6.6 | 15.95,16.6 12.7,16.6 12.2,16.1 USBKB.S1 | 15.95,16.6 21.95,16.6 23.95,14.6 26.2,14.6 26.2,11.1 U6.1 26.45,10.85 v27.45,9.85 | v28.45,5.6 27.2,5.6 26.7,5.1 C29.- | v36.2,5.1 34.45,5.1 C28.- | v13.2,45.85 12.45,45.85 12.2,46.1 U1.41_6
  Bottom 0.152: v47.95,50.6 58.2,40.35 59.7,40.35 J1.S2 | v27.45,9.85 v27.45,6.6 v28.45,5.6 28.45,5.1 v36.2,5.1 36.2,12.6 v37.2,13.6 | v13.2,45.85 15.95,43.1 v15.95,31.6
HSYNC  (via drill 0.25)
  Top 0.152: v47.45,47.1 45.95,47.1 45.95,49.35 X2.9 | v37.7,47.35 28.95,47.35 27.2,49.1 v23.7,49.1 | v23.2,45.85 21.45,44.1 20.95,44.1 U1.33
  Bottom 0.152: v47.45,47.1 48.2,47.85 48.2,48.35 43.2,53.35 37.7,53.35 v37.7,47.35 | v23.7,49.1 23.2,48.6 v23.2,45.85
INT  (via drill 0.25)
  Top 0.152: v49.2,48.1 49.45,48.1 49.95,48.6 49.95,49.35 X2.1 | v6.7,45.35 4.2,47.85 3.45,47.85 U1.5
  Bottom 0.152: v49.2,48.1 46.45,45.35 46.45,29.85 47.2,29.1 47.2,4.85 44.7,2.35 6.7,2.35 v6.7,45.35
IO0  (via drill 0.25)
  Top 0.152: v29.45,48.35 27.2,50.6 26.45,50.6 25.7,51.35 RESET.3 | v29.45,43.35 29.45,42.1 R7.2 | v23.2,36.6 20.95,36.6 U1.27
  Bottom 0.152: v29.45,43.35 v29.45,48.35 32.7,51.6 32.7,52.35 29.45,52.35 26.95,49.85 26.95,43.35 26.45,42.85 26.45,36.6 v23.2,36.6
LOUT  (via drill 0.25)
  Top 0.152: 50.45,9.35 53.95,9.35 AUDIO_CONN.2 | 50.45,9.35 v41.45,9.35 35.95,9.35 35.95,21.6 36.45,22.1 37.2,22.1 38.2,23.1 R20.1 | v41.45,17.1 43.45,17.1 43.7,17.35 C33.1 | 50.45,9.35 50.45,4.6 AUDIO_CONN.4
  Bottom 0.152: v41.45,9.35 v41.45,17.1
LRC  (via drill 0.25)
  Top 0.152: v50.2,26.35 47.2,29.35 45.7,29.35 45.45,29.6 U3.15 | v1.95,48.35 2.7,49.1 3.2,49.1 U1.4
  Bottom 0.152: v50.2,26.35 49.95,26.1 49.95,6.6 44.7,1.35 1.95,1.35 v1.95,48.35
MIDI_IN  (via drill 0.25)
  Top 0.152: v36.2,26.85 33.2,26.85 R16.1 30.2,24.1 22.45,24.1 v21.7,24.85 | v37.7,35.85 39.95,38.1 44.95,38.1 45.2,38.35 6N137S.6 | v19.7,34.1 16.45,34.1 16.45,35.1 U1.24
  Bottom 0.152: v36.2,26.85 37.7,28.35 v37.7,35.85 | v19.7,34.1 21.7,32.1 v21.7,24.85
MIDI_IN_SINK  (via drill 0.25)
  Top 0.152: 52.45,16.85 54.45,18.85 MIDI_IN_CONN.2 | 52.45,16.85 50.45,14.85 MIDI_IN_CONN.4 | v46.95,39.6 44.45,39.6 43.45,38.6 35.95,38.6 6N137S.3 | v49.2,36.35 50.2,35.35 D2.A | v48.2,21.1 52.45,16.85
  Bottom 0.152: 48.2,38.35 49.2,37.35 v49.2,36.35 | 48.2,38.35 v46.95,39.6 | 48.2,38.35 v48.2,21.1
MIDI_IN_SOURCE  (via drill 0.25)
  Top 0.152: v51.2,46.1 31.2,46.1 30.45,46.85 27.7,46.85 26.7,47.85 R15.2 | v61.2,13.85 61.2,12.1 61.7,12.1 MIDI_IN_CONN.3 61.95,12.1 64.7,12.1 MIDI_IN_CONN.5
  Bottom 0.152: v51.2,46.1 61.2,36.1 v61.2,13.85
MIDI_OUT  (via drill 0.25)
  Top 0.152: v23.45,18.85 23.7,19.1 33.2,19.1 34.2,20.1 R18.2 | v20.45,32.35 19.7,33.1 11.7,33.1 10.2,34.6 10.2,35.1 U1.19
  Bottom 0.152: v23.45,18.85 20.45,21.85 v20.45,32.35
MIDI_OUT_SINK
  Top 0.152: R18.1 32.2,22.1 32.95,22.1 33.45,22.6 33.45,25.35 49.7,25.35 50.2,24.85 | 50.2,24.85 54.45,29.1 MIDI_OUT_CONN.2 | 50.2,24.85 MIDI_OUT_CONN.4
MIDI_OUT_SOURCE
  Top 0.152: R17.2 34.45,23.1 36.2,24.85 47.7,24.85 50.45,22.1 MIDI_OUT_CONN.3 MIDI_OUT_CONN.5
N$1  (via drill 0.25)
  Top 0.152: v26.45,50.1 25.2,50.1 25.2,51.35 RESET.2 | v26.45,43.6 26.45,42.35 R1.1
  Bottom 0.152: v26.45,43.6 v26.45,50.1
N$2  (via drill 0.25)
  Top 0.152: v25.2,54.6 25.2,53.6 RESET.5 | v25.2,40.6 24.2,39.6 R6.2
  Bottom 0.152: v25.2,54.6 25.45,54.35 25.45,43.85 25.2,43.6 v25.2,40.6
N$3
  Top 0.152: R10.2 57.7,37.6 59.2,37.6 J1.B5
N$7  (via drill 0.25)
  Top 0.152: v43.45,31.6 45.2,31.6 U3.18 | v42.95,26.6 42.7,26.35 37.45,26.35 35.7,28.1 32.2,28.1 31.95,28.35 31.95,30.1 35.7,30.1 C8.1 | v40.2,4.6 38.7,4.6 38.45,4.85 C28.+
  Bottom 0.152: v43.45,31.6 42.95,31.1 v42.95,26.6 42.95,4.6 v40.2,4.6
N$8  (via drill 0.25)
  Top 0.152: R19.2 39.2,10.6 v38.2,10.6 | v38.2,28.85 39.45,28.85 U3.7
  Bottom 0.152: v38.2,28.85 v38.2,10.6
N$10  (via drill 0.25)
  Top 0.152: v31.45,46.6 53.95,46.6 55.45,48.1 POWER.2 | v30.7,23.85 29.95,23.1 14.95,23.1 13.95,22.1 J3.09 13.95,21.85 13.95,19.35 J3.11
  Bottom 0.152: v31.45,46.6 30.7,45.85 v30.7,23.85
N$16  (via drill 0.25)
  Top 0.152: v40.95,30.85 39.7,30.85 U3.4 | v41.45,23.85 41.95,23.35 43.7,23.35 C22.1
  Bottom 0.152: v40.95,30.85 41.45,30.35 v41.45,23.85
N$18  (via drill 0.25)
  Top 0.152: v40.95,32.1 39.7,32.1 U3.2 | v42.45,24.35 44.45,24.35 45.45,23.35 C22.2
  Bottom 0.152: v40.95,32.1 42.45,30.6 v42.45,24.35
N$30  (via drill 0.25)
  Top 0.152: v33.7,45.1 31.7,45.1 30.45,46.35 26.2,46.35 24.7,47.85 R15.1 | v34.2,41.6 34.7,41.1 35.7,41.1 6N137S.2 | v34.2,33.35 48.7,33.35 50.2,31.85 D2.C
  Bottom 0.152: v33.7,45.1 34.2,44.6 v34.2,41.6 v34.2,33.35
N$32  (via drill 0.25)
  Top 0.152: v40.45,21.6 40.45,20.35 R12.2 | v40.45,39.1 42.2,40.85 45.2,40.85 6N137S.7
  Bottom 0.152: v40.45,39.1 v40.45,21.6
N$38  (via drill 0.25)
  Top 0.152: v30.2,15.1 30.2,11.1 U6.4 | v31.2,38.1 31.2,39.1 C11.2
  Bottom 0.152: v30.2,15.1 31.2,16.1 v31.2,38.1
N$42
  Top 0.152: R9.1 55.95,36.35 57.7,36.35 57.7,34.85 57.95,34.6 59.2,34.6 J1.A5
OUTL  (via drill 0.25)
  Top 0.152: v40.95,24.35 40.45,24.35 40.45,23.35 R20.2 | v40.95,29.1 40.45,29.6 39.7,29.6 U3.6
  Bottom 0.152: v40.95,29.1 v40.95,24.35
PCLK  (via drill 0.25)
  Top 0.152: v44.45,48.1 44.95,48.1 44.95,49.35 X2.11 | v40.95,44.1 36.45,39.6 32.95,39.6 32.2,40.35 28.7,40.35 27.2,38.85 v27.2,37.6 | v23.2,35.85 22.95,35.6 19.95,35.6 19.7,35.85 19.7,36.35 14.7,36.35 13.7,35.35 U1.22
  Bottom 0.152: v44.45,48.1 40.95,48.1 v40.95,44.1 | v27.2,37.6 26.95,37.35 26.95,36.6 26.2,35.85 v23.2,35.85
PWM  (via drill 0.25)
  Top 0.152: v47.7,48.1 47.45,48.1 47.45,49.35 X2.6 | v7.45,39.1 3.95,42.6 3.45,42.6 U1.9
  Bottom 0.152: v47.7,48.1 44.95,45.35 44.95,5.6 42.2,2.85 7.45,2.85 v7.45,39.1
R5  (via drill 0.25)
  Top 0.152: v34.2,47.85 34.95,47.85 34.95,49.35 X2.31 | v33.2,31.1 32.7,30.6 v19.45,30.6 | v18.2,40.1 13.45,44.85 6.45,44.85 4.7,46.6 3.45,46.6 U1.6
  Bottom 0.152: v34.2,47.85 33.2,46.85 v33.2,31.1 | v19.45,30.6 18.2,31.85 v18.2,40.1
R6  (via drill 0.25)
  Top 0.152: v35.45,48.1 35.45,49.35 X2.30 | v4.45,46.1 3.7,45.35 3.45,45.35 U1.7
  Bottom 0.152: v35.45,48.1 35.2,48.35 35.2,52.6 32.7,55.1 21.2,55.1 21.2,54.35 18.45,51.6 4.45,51.6 v4.45,46.1
R7  (via drill 0.25)
  Top 0.152: v36.45,47.85 35.95,47.85 35.95,49.35 X2.29 | v32.2,15.6 23.45,15.6 21.2,17.85 v17.95,17.85 | v13.2,38.6 7.95,43.85 3.45,43.85 U1.8
  Bottom 0.152: v36.45,47.85 36.45,27.85 35.7,27.1 35.7,19.1 v32.2,15.6 | v17.95,17.85 13.2,22.6 v13.2,38.6
ROUT
  Top 0.152: AUDIO_CONN.5 64.7,1.85 61.95,1.85 AUDIO_CONN.3 61.7,1.85 61.7,4.85 55.7,10.85 42.95,10.85 40.95,12.85 37.2,12.85 | 37.2,12.85 36.45,13.6 36.45,21.6 39.7,21.6 40.2,22.1 41.95,22.1 C32.1 | 37.2,12.85 38.2,11.85 R19.1
SCL  (via drill 0.25)
  Top 0.152: v4.45,41.1 3.7,41.1 3.45,41.35 U1.10 | v3.95,31.1 7.2,27.85 17.2,27.85 17.95,27.1 J3.06 18.2,27.1 v20.95,27.1 | v34.2,52.1 48.95,52.1 48.95,49.35 X2.3 | v32.7,35.85 30.95,34.1 27.2,34.1 26.7,33.6 | 26.7,33.6 R14.2 26.45,33.35 | v24.95,31.1 v21.2,31.1 | 26.7,33.6 v25.95,34.35
  Bottom 0.152: v4.45,41.1 3.95,40.6 v3.95,31.1 | v34.2,52.1 32.7,50.6 v32.7,35.85 | v20.95,27.1 21.2,27.35 v21.2,31.1 | v24.95,31.1 25.95,32.1 v25.95,34.35
SDA  (via drill 0.25)
  Top 0.152: 2.45,39.85 2.95,39.85 3.2,40.1 U1.11 | 2.45,39.85 2.2,39.6 2.2,27.1 13.7,27.1 J3.05 | v31.95,51.6 48.45,51.6 48.45,49.35 X2.4 | v27.95,45.85 27.45,45.35 26.7,45.35 R13.2 26.45,45.35 25.95,45.35 v24.45,46.85 | 2.45,39.85 1.45,40.85 1.45,54.35 22.7,54.35 v23.2,53.85
  Bottom 0.152: v31.95,51.6 27.95,47.6 v27.95,45.85 | v23.2,53.85 24.45,52.6 v24.45,46.85
UART0_RXD  (via drill 0.25)
  Top 0.152: v25.95,15.1 27.45,15.1 27.45,11.1 U6.2 | v23.7,46.35 22.2,47.85 20.95,47.85 U1.36
  Bottom 0.152: v25.95,15.1 24.45,16.6 24.45,30.1 22.7,31.85 22.7,44.6 23.7,45.6 v23.7,46.35
UART0_TXD  (via drill 0.25)
  Top 0.152: v18.95,9.1 28.7,9.1 28.7,10.85 U6.3 | v19.45,48.35 20.2,49.1 20.7,49.1 U1.37
  Bottom 0.152: v18.95,9.1 16.45,11.6 16.45,15.35 18.45,17.35 18.45,31.1 17.7,31.85 17.7,46.6 v19.45,48.35
VNEG  (via drill 0.25)
  Top 0.152: v41.95,30.1 39.7,30.1 U3.5 | C23.1 v41.95,16.6
  Bottom 0.152: v41.95,16.6 v41.95,30.1
VSYNC  (via drill 0.25)
  Top 0.152: v23.2,54.6 23.7,55.1 50.45,55.1 50.45,48.6 49.45,47.6 46.45,47.6 46.45,49.35 X2.8 | v22.7,46.6 21.45,45.35 20.95,45.35 U1.34
  Bottom 0.152: v23.2,54.6 22.7,54.1 v22.7,46.6

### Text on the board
tNames: tulip.computer v4r6
tValues: Close
Measures: All dimensions in inches | Units: Inches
